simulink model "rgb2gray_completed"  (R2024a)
settings: Solver=VariableStepDiscrete  StartTime=0.0  StopTime=20  RelTol=1e-3  EnableMultiTasking=on
undefined symbols (not defined in the file or in its folder): Addsub_config, AXI4, Board, CMult_config, code, Constant_config, Convert_config, Evaluation, ffvc1156, gateway_in_config, gateway_out_config, hex2dec, Lite, Reinterpret_config, sysgen, UltraScale, xczu7ev, ZCU104, Zynq
libraries: hdlBasic x13, vmcUtilities x1

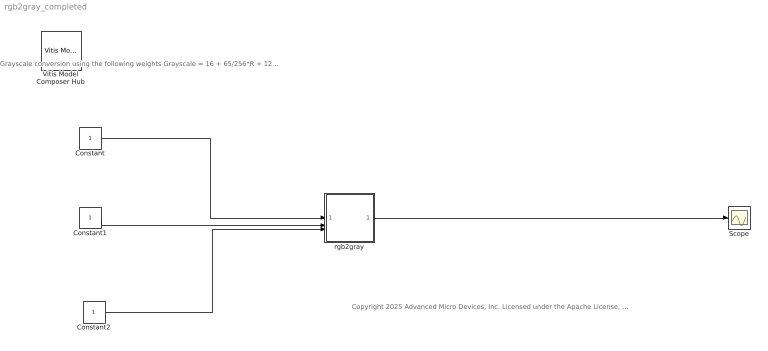
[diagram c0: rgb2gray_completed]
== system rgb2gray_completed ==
  note: Grayscale conversion using the following weights Grayscale = 16 + 65/256*R + 129/256*G + 25/256*B
  note: Copyright 2025 Advanced Micro Devices, Inc. Licensed under the Apache License, Version 2.0 (the "License"); you may not use this file except in compliance with the License. You may obtain a copy of the License at http://www.apache.org/licenses/LICENSE-2.0 Unless required by applicable law or agreed to in writing, software distributed under the License is distributed on an "AS IS" BASIS, WITHOUT WARRANTIES OR CONDITIONS OF ANY KIND, either express or implied. See the License for the specific language governing permissions and limitations under the License.
  Constant : Constant
  Constant1 : Constant
  Constant2 : Constant
  Scope : Scope
  Vitis Model Composer Hub : vmcUtilities/Vitis Model Composer Hub  Tag=genX  CodeGeneration=off  SubsystemName=rgb2gray  StartColumn=1  NumberOfColumns=1  TargetDirectory=./code  exportDesign=off  analyzeDesign=off  validateDesignOnHw=off  ExportType=HDL  IpVendor=xilinx.com  IpLibrary=hls  IpVersion=1.0  IpHWLanguage=Verilog  AieCompilerOptions={}  AieSimulatorOptions={}  CreateTestbench=off  TestbenchStackSize=10  RunRtlSim=off  RunCSim=off  RunAieSim=off  AieSimTimeout=50000  RunAieSimProfiling=off  LaunchVitisAnalyzer=off  PlotOutput=off  RunX86Sim=off  X86SimTimeout=10  GenHwImage=off  GenLibadfXo=off  GenHwValidationCode=off  PlatformType=Not Specified  HwSystemType=Baremetal  HwValidationTarget=hw  ProjDevice=Zynq UltraScale+ ZCU104 Evaluation Board (xczu7ev-ffvc1156-2-e)  ProjDevicePart=xczu7ev-ffvc1156-2-e  AIEType=None  SamplePeriod=-1  ClockFrequency=200  DataPathParallelism=1  xilinxfamily=zynquplus  part=xczu7ev  speed=-2-e  package=ffvc1156  directory=/home/amd/training/interface_synthesis/lab/ZCU104/model/./netlist_IP_Catalog/ip/rgb2gray/src  testbench=off  incr_netlist=off  synthesis_tool=Vivado  clock_wrapper=Clock Enables  dbl_ovrd=According to Block Masks  dcm_input_clock_period=10  sysclk_period=10  simulink_period=1  eval_field=0  IPInfoJsonString="{\"HDLSubsystem\":{\"SubsystemName\":\"rgb2gray\",\"IPName\":\"rgb2gray\",\"IPLibrary\":\"VMC\",\"IPVendor\":\"User Company\",\"IPVersion\":\"1.0\",\"TargetDirectory\":\"/home/amd/training/interface_synthesis/lab/ZCU104/model/./netlist_IP_Catalog\",\"SubsystemDir\":\"/home/amd/training/interface_synthesis/lab/ZCU104/model/./netlist_IP_Catalog/ip/rgb2gray\"}}"  LogFileName=''  NThreads=4
  rgb2gray : Subsystem
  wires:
  Constant/1 -> rgb2gray/1(In1)
  Constant1/1 -> rgb2gray/2(In2)
  Constant2/1 -> rgb2gray/3(In3)
  rgb2gray/1(Out1) -> Scope/1

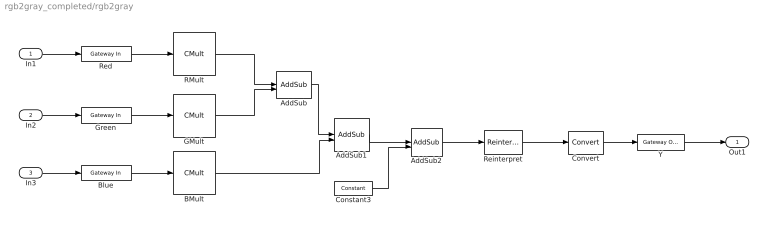
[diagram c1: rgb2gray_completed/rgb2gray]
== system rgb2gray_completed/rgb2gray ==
  In1 : Inport
  In2 : Inport  Port=2
  In3 : Inport  Port=3
  AddSub : hdlBasic/AddSub  mode=Addition  use_carryin=off  use_carryout=off  en=off  latency=1  precision=Full  arith_type=Unsigned  n_bits=8  bin_pt=2  quantization=Truncate  overflow=Wrap  use_behavioral_HDL=on  hw_selection=Fabric  pipelined=off  use_rpm=on  XmcBlockStatus=1  maskContainerNames=tabcontainer1  block_type=addsub  block_config=sysgen:Addsub_config
  AddSub1 : hdlBasic/AddSub  mode=Addition  use_carryin=off  use_carryout=off  en=off  latency=0  precision=Full  arith_type=Unsigned  n_bits=8  bin_pt=2  quantization=Truncate  overflow=Wrap  use_behavioral_HDL=on  hw_selection=Fabric  pipelined=off  use_rpm=on  XmcBlockStatus=1  maskContainerNames=tabcontainer1  block_type=addsub  block_config=sysgen:Addsub_config
  AddSub2 : hdlBasic/AddSub  mode=Addition  use_carryin=off  use_carryout=off  en=off  latency=1  precision=Full  arith_type=Unsigned  n_bits=8  bin_pt=2  quantization=Truncate  overflow=Wrap  use_behavioral_HDL=on  hw_selection=Fabric  pipelined=off  use_rpm=on  XmcBlockStatus=1  maskContainerNames=tabcontainer1  block_type=addsub  block_config=sysgen:Addsub_config
  BMult : hdlBasic/CMult  const=25  gui_display_data_type=Fixed-point  const_n_bits=8  const_bin_pt=0  float_type=Single  exp_bits=8  fraction_bits=24  en=off  latency=1  precision=Full  arith_type="Signed  (2's comp)"  n_bits=8  bin_pt=6  quantization="Round  (unbiased: +/- Inf)"  overflow=Wrap  use_behavioral_HDL=off  mem_type=Distributed RAM  pipeline=off  use_rpm=on  placement_style=Rectangular Shape  XmcBlockStatus=1  maskContainerNames=tabcontainer1  block_type=cmult  block_config=sysgen:CMult_config
  Blue : hdlBasic/Gateway In  gui_display_data_type=Fixed-point  arith_type=Unsigned  n_bits=8  bin_pt=0  preci_type=Single  exp_width=8  frac_width=24  rows=1  columns=1  quantization="Round  (unbiased: +/- Inf)"  overflow=Saturate  period=1  UseAsADC=off  ADCChannel='1'  interface=AXI4-Lite  automatic_assignment=on  address_offset=hex2dec('00')  intf_name=''  intf_description='Blue'  default_value=0  timing_constraint=None  locs_specified=off  LOCs={}  io_standard={}  inherit_from_input=off  hdl_port=on  XmcBlockStatus=1  maskContainerNames=group4  block_type=gatewayin  block_config=sysgen:gateway_in_config  block_width_w=590  block_height_w=620  block_width=640  block_height=850
  Constant3 : hdlBasic/Constant  const=16*256  gui_display_data_type=Fixed-point  arith_type=Unsigned  n_bits=16  bin_pt=0  preci_type=Single  exp_width=8  frac_width=24  explicit_period=off  period=1  XmcBlockStatus=1  maskContainerNames=tabcontainer1  block_type=constant  block_config=sysgen:Constant_config
  Convert : hdlBasic/Convert  gui_display_data_type=Fixed-point  arith_type=Unsigned  n_bits=8  bin_pt=0  float_type=Single  exp_bits=8  fraction_bits=24  quantization="Round  (unbiased: Even Values)"  overflow=Saturate  en=off  latency=0  pipeline=off  XmcBlockStatus=1  maskContainerNames=group2  block_type=convert  block_config=sysgen:Convert_config  block_width=595  block_height=885
  GMult : hdlBasic/CMult  const=129  gui_display_data_type=Fixed-point  const_n_bits=8  const_bin_pt=0  float_type=Single  exp_bits=8  fraction_bits=24  en=off  latency=0  precision=Full  arith_type="Signed  (2's comp)"  n_bits=8  bin_pt=6  quantization="Round  (unbiased: +/- Inf)"  overflow=Wrap  use_behavioral_HDL=off  mem_type=Distributed RAM  pipeline=off  use_rpm=on  placement_style=Rectangular Shape  XmcBlockStatus=1  maskContainerNames=tabcontainer1  block_type=cmult  block_config=sysgen:CMult_config
  Green : hdlBasic/Gateway In  gui_display_data_type=Fixed-point  arith_type=Unsigned  n_bits=8  bin_pt=0  preci_type=Single  exp_width=8  frac_width=24  rows=1  columns=1  quantization="Round  (unbiased: +/- Inf)"  overflow=Saturate  period=1  UseAsADC=off  ADCChannel='1'  interface=AXI4-Lite  automatic_assignment=on  address_offset=hex2dec('02')  intf_name=''  intf_description='Green'  default_value=0  timing_constraint=None  locs_specified=off  LOCs={}  io_standard={}  inherit_from_input=off  hdl_port=on  XmcBlockStatus=1  maskContainerNames=group4  block_type=gatewayin  block_config=sysgen:gateway_in_config  block_width_w=590  block_height_w=620  block_width=640  block_height=850
  RMult : hdlBasic/CMult  const=65  gui_display_data_type=Fixed-point  const_n_bits=8  const_bin_pt=0  float_type=Single  exp_bits=8  fraction_bits=24  en=off  latency=0  precision=Full  arith_type="Signed  (2's comp)"  n_bits=8  bin_pt=6  quantization="Round  (unbiased: +/- Inf)"  overflow=Wrap  use_behavioral_HDL=off  mem_type=Distributed RAM  pipeline=off  use_rpm=on  placement_style=Rectangular Shape  XmcBlockStatus=1  maskContainerNames=tabcontainer1  block_type=cmult  block_config=sysgen:CMult_config
  Red : hdlBasic/Gateway In  gui_display_data_type=Fixed-point  arith_type=Unsigned  n_bits=8  bin_pt=0  preci_type=Single  exp_width=8  frac_width=24  rows=1  columns=1  quantization="Round  (unbiased: +/- Inf)"  overflow=Saturate  period=1  UseAsADC=off  ADCChannel='1'  interface=AXI4-Lite  automatic_assignment=on  address_offset=hex2dec('00')  intf_name=''  intf_description='Red'  default_value=0  timing_constraint=None  locs_specified=off  LOCs={}  io_standard={}  inherit_from_input=off  hdl_port=on  XmcBlockStatus=1  maskContainerNames=group4  block_type=gatewayin  block_config=sysgen:gateway_in_config  block_width_w=590  block_height_w=620  block_width=640  block_height=850
  Reinterpret : hdlBasic/Reinterpret  force_arith_type=off  arith_type=Unsigned  force_bin_pt=on  bin_pt=8  XmcBlockStatus=1  maskContainerNames=group1  block_type=reinterpret  block_config=sysgen:Reinterpret_config
  Y : hdlBasic/Gateway Out  inherit_from_input=off  hdl_port=on  rows=1  columns=1  UseAsDAC=off  DACChannel='1'  interface=AXI4-Lite  automatic_assignment=on  address_offset=hex2dec('00')  intf_name=''  intf_description='Luminance'  timing_constraint=None  locs_specified=off  LOCs={}  io_standard={}  XmcBlockStatus=1  maskContainerNames=group4  block_type=gatewayout  block_config=sysgen:gateway_out_config  block_width_w=590  block_height_w=620  block_width=620  block_height=750
  Out1 : Outport
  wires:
  Blue/1 -> BMult/1
  AddSub2/1 -> Reinterpret/1
  Green/1 -> GMult/1
  In3/1 -> Blue/1
  In2/1 -> Green/1
  GMult/1 -> AddSub/2
  Constant3/1 -> AddSub2/2
  Y/1 -> Out1/1
  In1/1 -> Red/1
  AddSub/1 -> AddSub1/1
  AddSub1/1 -> AddSub2/1
  Reinterpret/1 -> Convert/1
  Convert/1 -> Y/1
  RMult/1 -> AddSub/1
  Red/1 -> RMult/1
  BMult/1 -> AddSub1/2
